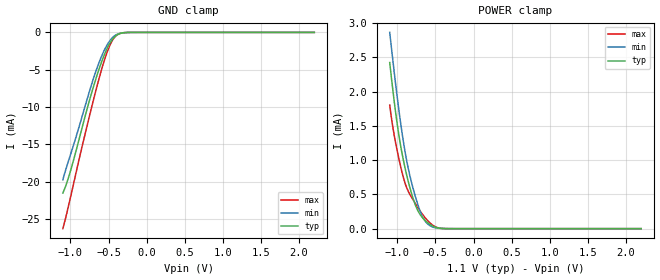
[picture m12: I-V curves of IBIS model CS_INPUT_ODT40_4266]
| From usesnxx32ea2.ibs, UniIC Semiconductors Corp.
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| CS_INPUT_ODT40_4266 (with 40ohm ODT, 3200-4266Mbps)
[Model]   CS_INPUT_ODT40_4266
Model_type   Input
Vinl = 110.833mV
Vinh = 255.833mV
|   typ   min   max
|C_comp   0.631pF   0.581pF   0.698pF
C_comp_power_clamp   0.3155pF   0.2905pF   0.3490pF
C_comp_gnd_clamp   0.3155pF   0.2905pF   0.3490pF
| Note: C_comp changes when the ODT circuit is enabled.
[Model Spec]
| Input threshold voltage corners
Vinl   0.1108V   0.1042V   0.1225V
Vinh   0.2558V   0.2492V   0.2675V
| Dynamic Overshoot Parameters from LPDDR4 Specification
D_overshoot_ampl_h   0.30   NA   NA
D_overshoot_ampl_l   0.30   NA   NA
D_overshoot_area_h   0.1n   NA   NA
D_overshoot_area_l   0.1n   NA   NA
[Voltage Range]   1.1000V   1.0600V   1.1700V
[POWER Clamp Reference]   1.1000V   1.0600V   1.1700V
| Junction Temperature (Ambient temp is 35C typ 95C min -40C max)
[Temperature Range]   50.0   110.0   -40.0
[Add Submodel]
| Submodel Name   Mode
40ohm_ODT_4266   Non-Driving
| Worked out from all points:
|   GND clamp passes 1 mA (typ) near -0.45 V on its own axis
|   POWER clamp passes 1 mA (typ) near -0.92 V on its own axis
[GND Clamp]
|   Voltage   I(typ)   I(min)   I(max)
-1.1V     -21.5mA    -19.73mA   -26.28mA
-1.05V    -20.21mA   -18mA      -24.3mA
-1.001V   -18.6mA    -16.41mA   -22.14mA
-756.8mV  -9.322mA   -8.095mA   -11.46mA
-674.3mV  -6.479mA   -5.435mA   -8.089mA
-611.6mV  -4.527mA   -3.692mA   -5.688mA
-558.8mV  -3.075mA   -2.45mA    -3.855mA
-496.1mV  -1.68mA    -1.302mA   -2.043mA
-446.6mV  -895.4uA   -681.7uA   -1.019mA
-390.5mV  -360.6uA   -270.9uA   -358.3uA
-215.6mV  -4.605uA   -4.495uA   -2.165uA
2.2V      0A         0A         0A
[POWER Clamp]
|   Voltage   I(typ)   I(min)   I(max)
-1.1V     2.422mA    2.862mA    1.802mA
-1.041V   1.851mA    2.277mA    1.359mA
-991.1mV  1.446mA    1.826mA    1.078mA
-931.7mV  1.06mA     1.348mA    793.2uA
-872.3mV  758.1uA    963.8uA    583.4uA
-789.8mV  428.8uA    572.2uA    413.9uA
-723.8mV  247.8uA    326.1uA    295.1uA
-654.5mV  141uA      142.6uA    185.5uA
-591.8mV  77.55uA    58.75uA    105.2uA
-499.4mV  21.2uA     12.49uA    27.17uA
-400.4mV  2.408uA    1.511uA    2.096uA
2.2V      0A         0A         0A
